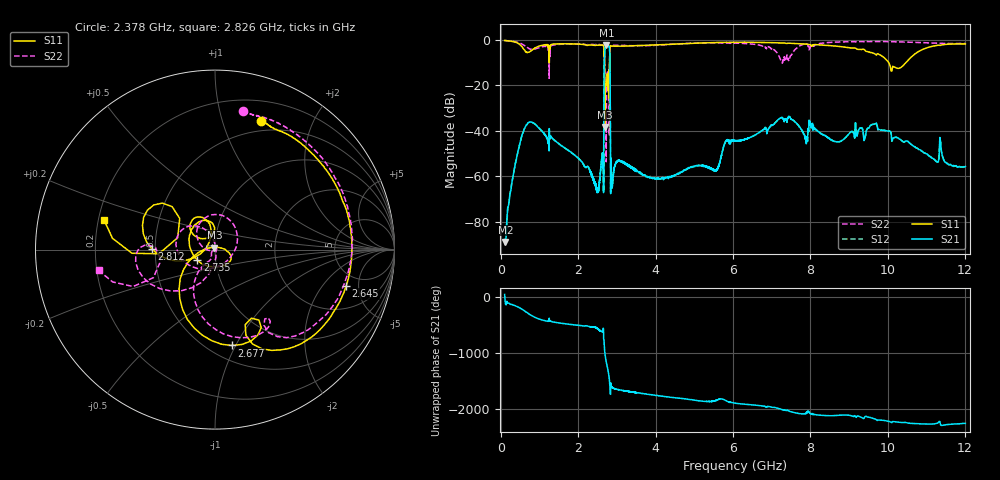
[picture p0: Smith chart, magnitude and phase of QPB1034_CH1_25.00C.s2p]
! TDS: k:\Engsetup\Winsaw\QPB1034_ALL
! Channel 1
! Ports=1 2
! seg 1=100.000000 1100.000000 51
! seg 2=1101.000000 1301.000000 201
! seg 3=1302.000000 2302.000000 101
! seg 4=2303.000000 3503.000000 1201
! seg 5=3504.000000 5204.000000 171
! seg 6=5205.000000 6405.000000 1201
! seg 7=6406.000000 8506.000000 211
! seg 8=8507.000000 12007.000000 176
! Points=3313
! FailCode=0
! Topology=ALL_SE(12)
!VNA Cal loaded =QPB1034_ALL_25C
!PS1(V)= 5.000
!PS(mA)= 0.232
!PS2(V)= 0.630
!PS(mA)= -0.002
!PS3(V)= 0.630
!PS(mA)= -0.001
!PS4(V)= 1.170
!PS(mA)= -0.001
!Temp (C)= 25.00
# MHz S DB R 50
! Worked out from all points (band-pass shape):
!   3313 points, 100 MHz to 12.01 GHz, reference 50 ohm
!   highest |S21| = -2.26 dB at 2.73 GHz (marker M1); lowest = -89.0 dB at 120 MHz (marker M2)
!   |S21| within 3 dB of the highest: 2.685 GHz to 2.814 GHz (129.5 MHz wide, 4.71 % of centre)
!   lowest |S11| = -38.4 dB at 2.693 GHz (marker M3), VSWR 1.02, Z = 49.7 + j1.15 ohm
!   |S11| at or under -10 dB: 2.684 GHz to 2.811 GHz (126.6 MHz wide, 4.61 % of centre); 2.820265 GHz to 2.823021 GHz (2.756 MHz wide, 0.0977 % of centre); 10.02 GHz to 10.48 GHz (453.2 MHz wide, 4.42 % of centre)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
!   |S22| runs from -53.7 to -0.3 dB; largest |S21 - S12| = 0.0039
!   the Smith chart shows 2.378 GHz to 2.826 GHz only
!   S11 on the Smith chart (normalised r, x): 2.378 GHz: 0.39, +1.34; 2.645 GHz: 3.74, -3.57; 2.677 GHz: 0.64, -0.97; 2.735 GHz: 0.82, -0.09; 2.812 GHz: 0.48, +0.00; 2.826 GHz: 0.22, +0.12
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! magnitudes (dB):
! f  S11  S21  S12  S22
! 100 MHz  -0.3  -87.8  -88.0  -0.3
! 120 MHz  -0.3  -89.0  -90.8  -0.3
! 240 MHz  -0.6  -67.8  -67.0  -0.5
! 500 MHz  -2.2  -45.3  -45.2  -1.5
! 1.1 GHz  -2.3  -40.8  -40.9  -2.9
! 2.378 GHz  -2.4  -60.5  -60.6  -2.1
! 2.434 GHz  -2.5  -62.8  -62.8  -2.1
! 2.645 GHz  -2.4  -54.6  -54.7  -2.4
! 2.677 GHz  -5.3  -9.1  -9.1  -5.6
! 2.693 GHz  -38.4  -3.4  -3.4  -20.3
! 2.713 GHz  -19.6  -2.6  -2.6  -35.3
! 2.73 GHz  -19.9  -2.3  -2.3  -32.8
! 2.735 GHz  -18.9  -2.3  -2.3  -23.9
! 2.812 GHz  -9.1  -4.4  -4.4  -9.4
! 2.826 GHz  -3.9  -15.5  -15.5  -3.6
! 2.85 GHz  -2.7  -52.3  -52.5  -2.4
! 2.88 GHz  -2.8  -65.0  -64.6  -2.4
! 3.042 GHz  -2.8  -53.4  -53.3  -2.4
! 5.406 GHz  -1.3  -56.4  -56.5  -1.3
! 7.346 GHz  -1.5  -35.2  -35.2  -8.7
! 10.25 GHz  -12.5  -43.1  -43.1  -0.9
! 12.01 GHz  -1.8  -55.7  -55.9  -1.6
